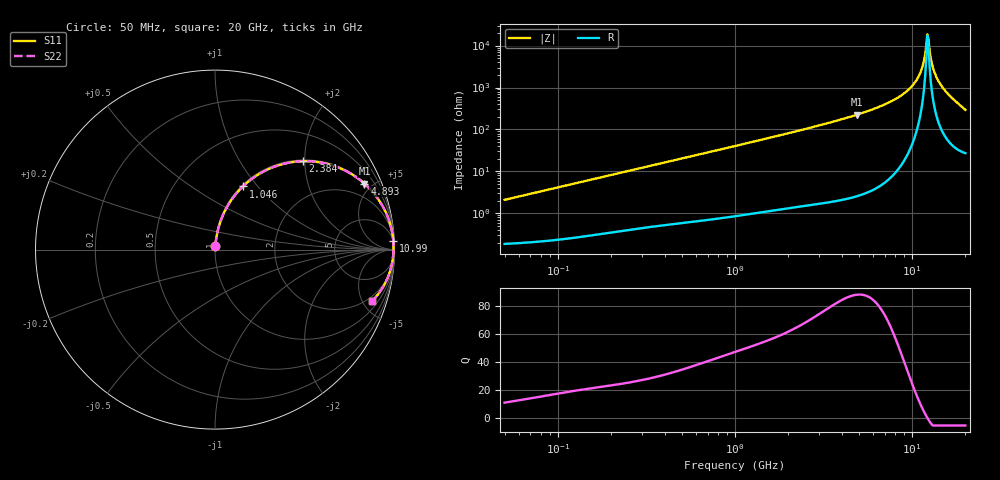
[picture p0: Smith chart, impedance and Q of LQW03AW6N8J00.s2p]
!Murata Part Number: LQW03AW6N8J00
!These Parameters are Measured in Series Mode Connection
!  o--[Z]--o
!Port1  Port2
!  o-------o
!Freq. Start=50[MHz] Stop=20[GHz], 401[Steps]
# Hz S RI R 50
!Freq.(Hz) S11(Real) S11(Imag) S21(Real) S21(Imag) S12(Real) S12(Imag) S22(Real) S22(Imag)
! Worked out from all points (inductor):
!   401 points, 50 MHz to 20 GHz, reference 50 ohm
!   read as one part in series: L = 6.63 nH near 51.52 MHz
!   highest Q = 88 at 4.893 GHz (marker M1), where L = 7.33 nH
!   self-resonance near 12.2 GHz
!   S11 on the Smith chart (normalised r, x): 50 MHz: 1.00, +0.04; 1.046 GHz: 1.02, +0.84; 2.384 GHz: 1.03, +1.95; 4.893 GHz: 1.05, +4.51; 10.99 GHz: 4, +40; 20 GHz: 1.54, -5.84
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5e7  0.00229 0.0208  0.9977 -0.0208  0.9977 -0.0208  0.00229 0.0208
1.364002e8  0.00588 0.0558  0.9941 -0.0558  0.9941 -0.0558  0.00588 0.0558
3.721004e8  0.0268 0.1459  0.9732 -0.1459  0.9732 -0.1459  0.0268 0.1459
1e9  0.1441 0.3408  0.8559 -0.3408  0.8559 -0.3408  0.1441 0.3408
1.045961e9  0.1552 0.3518  0.8448 -0.3518  0.8448 -0.3518  0.1552 0.3518
2.383959e9  0.4884 0.4924  0.5116 -0.4924  0.5116 -0.4924  0.4884 0.4924
2.728004e9  0.5594 0.4895  0.4406 -0.4895  0.4406 -0.4895  0.5594 0.4895
4.89267e9  0.8326 0.3677  0.1674 -0.3677  0.1674 -0.3677  0.8326 0.3677
7.442007e9  0.949 0.2126  0.051 -0.2126  0.051 -0.2126  0.949 0.2126
9.457416e9  0.9832 0.1142  0.0168 -0.1142  0.0168 -0.1142  0.9832 0.1142
1.034674e10  0.9904 0.0757  0.00964 -0.0757  0.00964 -0.0757  0.9904 0.0757
1.098561e10  0.9933 0.0494  0.00665 -0.0494  0.00665 -0.0494  0.9933 0.0494
1.149051e10  0.9946 0.0293  0.00538 -0.0293  0.00538 -0.0293  0.9946 0.0293
1.201863e10  0.995 0.00878  0.005 -0.00878  0.005 -0.00878  0.995 0.00878
1.220001e10  0.9949 0.00183  0.00508 -0.00183  0.00508 -0.00183  0.9949 0.00183
1.238412e10  0.9947 -0.00518  0.00527 0.00518  0.00527 0.00518  0.9947 -0.00518
1.257102e10  0.9944 -0.0123  0.00557 0.0123  0.00557 0.0123  0.9944 -0.0123
1.314879e10  0.9928 -0.0339  0.00718 0.0339  0.00718 0.0339  0.9928 -0.0339
1.354865e10  0.9911 -0.0486  0.00889 0.0486  0.00889 0.0486  0.9911 -0.0486
1.417136e10  0.9875 -0.0714  0.0125 0.0714  0.0125 0.0714  0.9875 -0.0714
1.621653e10  0.9666 -0.1457  0.0334 0.1457  0.0334 0.1457  0.9666 -0.1457
2e10  0.8747 -0.2879  0.1253 0.2879  0.1253 0.2879  0.8747 -0.2879
